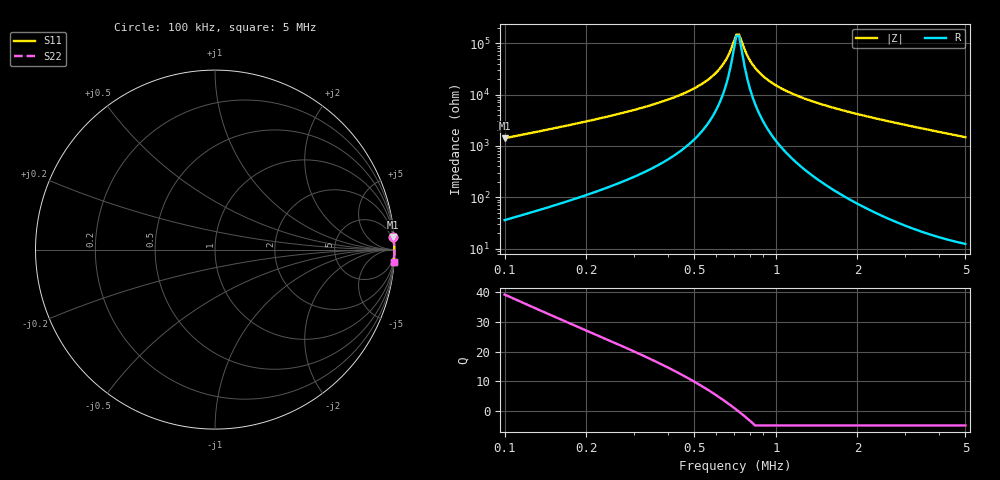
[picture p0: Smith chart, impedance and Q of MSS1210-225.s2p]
# MHz S MA R 50
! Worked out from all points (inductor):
!   172 points, 100 kHz to 5 MHz, reference 50 ohm
!   read as one part in series: L = 2.2 mH near 100 kHz
!   highest Q = 39.3 at 100 kHz (marker M1), where L = 2.24 mH
!   self-resonance near 715.2 kHz
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0.1  0.9957 4.1  0.07067 -84.5  0.07067 -84.5  0.9957 4.1
0.1475379  0.9975 2.7  0.0469 -85.5  0.0469 -85.5  0.9975 2.7
0.207939  0.9983 1.8  0.03188 -86.0  0.03188 -86.0  0.9983 1.8
0.4738205  0.9992 0.5  0.008748 -84.3  0.008748 -84.3  0.9992 0.5
0.568981  0.9993 0.3  0.004901 -81.3  0.004901 -81.3  0.9993 0.3
0.6094026  0.9993 0.2  0.003516 -78.4  0.003516 -78.4  0.9993 0.2
0.6526957  0.9993 0.1  0.002169 -71.8  0.002169 -71.8  0.9993 0.1
0.6832533  0.9993 0.1  0.00132 -60.0  0.00132 -60.0  0.9993 0.1
0.7152416  0.9994 0.0  0.0006834 -19.6  0.0006834 -19.6  0.9994 0.0
0.731793  0.9994 -0.0  0.0006765 19.7  0.0006765 19.7  0.9994 -0.0
0.783781  0.9994 -0.1  0.001716 68.9  0.001716 68.9  0.9994 -0.1
0.8204757  0.9994 -0.1  0.002592 76.4  0.002592 76.4  0.9994 -0.1
0.8588884  0.9994 -0.2  0.003496 80.1  0.003496 80.1  0.9994 -0.2
0.9199055  0.9994 -0.3  0.004881 83.0  0.004881 83.0  0.9994 -0.3
1.031385  0.9994 -0.4  0.007258 85.3  0.007258 85.3  0.9994 -0.4
1.210512  0.9994 -0.6  0.01076 86.7  0.01076 86.7  0.9994 -0.6
1.453628  0.9994 -0.9  0.01511 87.3  0.01511 87.3  0.9994 -0.9
1.745569  0.9994 -1.1  0.01998 87.6  0.01998 87.6  0.9994 -1.1
2.575376  0.999 -1.9  0.03276 87.4  0.03276 87.4  0.999 -1.9
3.388961  0.9986 -2.6  0.04465 86.9  0.04465 86.9  0.9986 -2.6
4.260117  0.9979 -3.3  0.05707 86.2  0.05707 86.2  0.9979 -3.3
5  0.9972 -3.9  0.06748 85.7  0.06748 85.7  0.9972 -3.9
